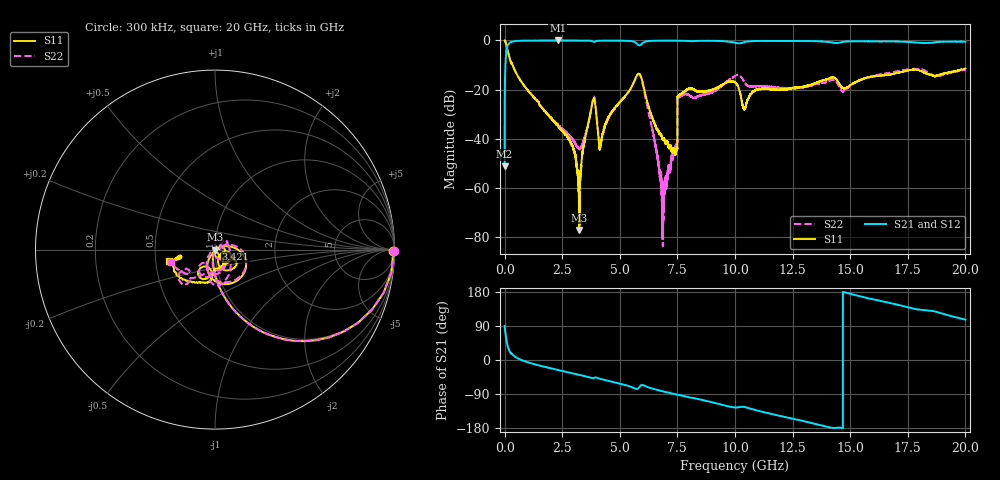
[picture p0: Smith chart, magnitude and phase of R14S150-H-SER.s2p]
!{R14S150}
!Johanson Technology Inc.
!www.johansontechnology.com
!Test Board Conditions:
!Substrate Type  RO4350B
!Substrate Thickness  20 mil
!Substrate Dk  3.66
!TL Type: GCPW
!TL Trace Width  36 mil
!TL Gap  12 mil
!Electrode orientation  Horizontal
!DUT TOPOLOGY	SERIES
!Mounting Pad LxW  26x36 mil
! Created Wed Nov 25 17:33:21 2020
! 2 Port Network Data from SP1.SP block
! freq  magS11  angS11  magS21  angS21  magS12  angS12  magS22  angS22
# khz S ma R 50
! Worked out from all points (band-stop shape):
!   20001 points, 300 kHz to 20 GHz, reference 50 ohm
!   highest |S21| = -0.01 dB at 2.306 GHz (marker M1); lowest = -51.1 dB at 300 kHz (marker M2)
!   |S21| within 3 dB of the highest: 106.3 MHz to end of sweep
!   lowest |S11| = -77.0 dB at 3.237 GHz (marker M3), VSWR 1.00, Z = 50 + j0.0133 ohm
!   |S11| at or under -10 dB: 342.1 MHz to end of sweep
!   |S22| runs from -83.7 to 0.0 dB; largest |S21 - S12| = 0.019
!   S11 on the Smith chart (normalised r, x): 300 kHz: open; 3.421 GHz: 1.01, +0.01; 20 GHz: 0.59, -0.08
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300  0.9937 -0.3  0.002786 90.1  0.002833 89.4  0.9977 -0.3
103300  0.7146 -45.6  0.6962 44.4  0.6978 44.3  0.7153 -45.5
200300  0.4662 -64.5  0.8823 25.3  0.8823 25.2  0.4674 -64.5
2306300  0.01865 -117.7  0.9985 -26.1  0.9967 -26.2  0.0197 -105.0
2958300  0.007047 -135.3  0.9974 -35.1  0.9965 -35.1  0.009647 -86.5
3237300  0.0001405 109.3  0.9966 -39.0  0.9957 -38.9  0.006388 -47.9
3334300  0.003182 47.7  0.9958 -40.3  0.9957 -40.3  0.00691 -21.2
3421300  0.006889 45.3  0.9947 -41.6  0.9944 -41.5  0.008948 1.2
3839300  0.06075 -11.0  0.9475 -48.2  0.9471 -48.2  0.06484 -13.3
4166300  0.007257 -10.2  0.991 -50.0  0.9917 -50.0  0.007779 -23.5
5823300  0.212 -52.3  0.7978 -73.4  0.7982 -73.4  0.2044 -50.0
6667300  0.0148 -102.9  0.9883 -79.7  0.9877 -79.7  0.003188 167.5
6805300  0.0115 -94.9  0.9899 -81.8  0.9893 -81.8  0.001197 118.8
6930300  0.01001 -92.9  0.9901 -83.6  0.9902 -83.6  0.0009111 8.1
7398300  0.00481 -61.7  0.9905 -90.2  0.9906 -90.2  0.006554 -62.1
7600300  0.07907 -55.7  0.9864 -93.0  0.9864 -93.0  0.07201 44.1
1.00003e7  0.1413 -53.9  0.9002 -125.2  0.9008 -125.2  0.1904 -74.6
1.04033e7  0.04017 -39.3  0.9244 -123.9  0.9238 -124.0  0.1441 -101.2
1.09763e7  0.09965 -21.7  0.9768 -133.5  0.9738 -133.6  0.1165 -76.6
1.33343e7  0.1263 -93.1  0.9702 -166.5  0.9726 -166.6  0.1214 -69.8
1.66673e7  0.1998 -114.4  0.9576 151.2  0.9507 151.2  0.2183 -129.6
2e7  0.2661 -166.4  0.94 106.4  0.9403 106.6  0.257 -164.1
